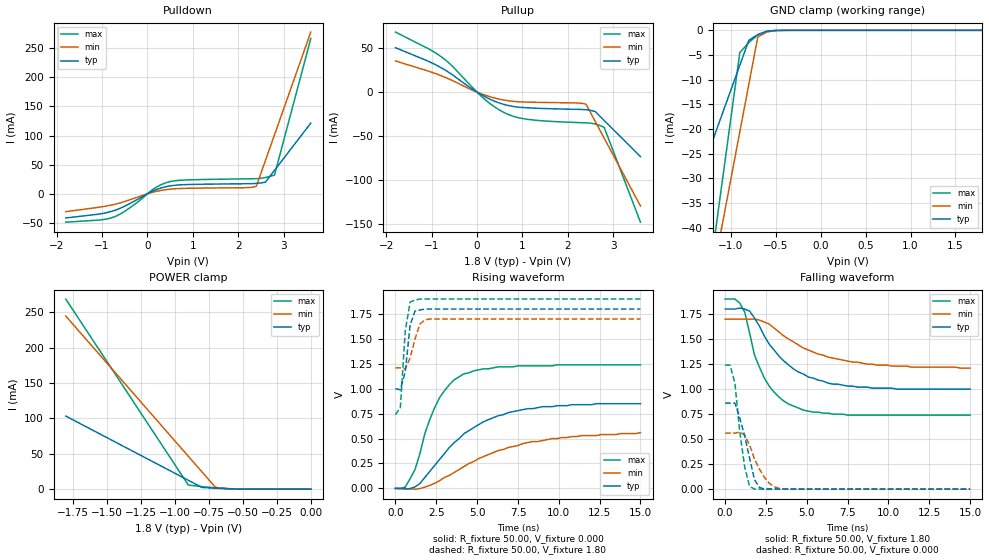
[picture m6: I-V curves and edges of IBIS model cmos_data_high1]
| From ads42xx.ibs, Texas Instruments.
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|   Model cmos_data_high1
[Model]   cmos_data_high1
Model_type   3-state
Polarity   Non-Inverting
Vmeas = 1.0000V
Enable   Active-High
C_comp   5.00pF   2.00pF   8.00pF
[Temperature Range]   25.00   0.12k   -40.00
[Voltage Range]   1.80V   1.70V   1.90V
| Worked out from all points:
|   slope of the pulldown table from 0 to 0.27 V, typ, clamps not added: 29.2 ohm
|   slope of the pullup table from 0 to 0.27 V, typ, clamps not added: 35.5 ohm
|   GND clamp passes 1 mA (typ) near -0.71 V on its own axis
|   POWER clamp passes 1 mA (typ) near -0.67 V on its own axis
|   rising waveform, R_fixture 50.00, V_fixture 0.000: 20-80 % time 3.45ns typ, 4.74ns min, 1.75ns max; typ from 0 V to 0.85 V
|   rising waveform, R_fixture 50.00, V_fixture 1.80: 20-80 % time 317ps typ, 509ps min, 328ps max; typ from 1 V to 1.8 V
|   falling waveform, R_fixture 50.00, V_fixture 1.80: 20-80 % time 2.59ns typ, 3.6ns min, 1.64ns max; typ from 1.8 V to 1 V
|   falling waveform, R_fixture 50.00, V_fixture 0.000: 20-80 % time 755ps typ, 964ps min, 534ps max; typ from 0.86 V to 0 V
[Pulldown]
| voltage   I(typ)   I(min)   I(max)
-1.8V     -41.57mA   -30.74mA   -48.79mA
-1V       -34mA      -22.32mA   -44.53mA
-700mV    -27.96mA   -17.7mA    -38.73mA
-400mV    -17.21mA   -10.58mA   -24.77mA
200mV     7.39mA     4.22mA     11.56mA
500mV     13.57mA    7.94mA     20.94mA
900mV     15.87mA    9.45mA     23.85mA
2.2V      17.23mA    10.57mA    25.67mA
2.4V      17.81mA    12.94mA    25.96mA
2.6V      19.98mA    57.06mA    27.9mA
2.8V      40.26mA    101.2mA    32.1mA
3.6V      121.4mA    277.7mA    266.5mA
[Pullup]
| voltage   I(typ)   I(min)   I(max)
-1.8V     50.62mA    35.54mA    68.37mA
-800mV    28.07mA    18.87mA    40.65mA
-600mV    21.79mA    14.59mA    32.3mA
100mV     -3.08mA    -2mA       -4.97mA
400mV     -10.55mA   -6.83mA    -17.27mA
600mV     -14.02mA   -9.04mA    -23.26mA
800mV     -16.26mA   -10.45mA   -27.47mA
1.1V      -17.71mA   -11.24mA   -30.76mA
2.4V      -19.9mA    -13.64mA   -34.86mA
2.6V      -21.9mA    -32.94mA   -36.12mA
2.8V      -32.16mA   -52.24mA   -39.99mA
3.6V      -73.2mA    -129.4mA   -147.8mA
[GND_clamp]
| voltage   I(typ)   I(min)   I(max)
-1.8V     -52.44mA   -107mA     -124.6mA
-1.6V     -42.36mA   -87.76mA   -97.9mA
-1.5V     -37.32mA   -78.16mA   -84.56mA
-1.2V     -22.2mA    -49.36mA   -44.54mA
-1.1V     -17.16mA   -39.76mA   -31.2mA
-1V       -12.12mA   -30.16mA   -17.86mA
-900mV    -7.08mA    -20.56mA   -4.52mA
-800mV    -2.04mA    -10.96mA   -2.47mA
-700mV    -860uA     -1.36mA    -940uA
-600mV    -210uA     -340uA     -160uA
-400mV    -1.56uA    -9.52uA    -280nA
1.8V      21.86pA    20.03nA    16.21pA
[POWER_clamp]
| voltage   I(typ)   I(min)   I(max)
-1.8V     103.3mA    244.7mA    268.7mA
-900mV    12.58mA    46.54mA    5.82mA
-800mV    2.5mA      24.52mA    3.54mA
-700mV    1.23mA     2.5mA      1.83mA
-500mV    85.21uA    200uA      92.55uA
0V        21.86pA    600pA      19.03pA
[Ramp]
| variable   typ   min   max
dV/dt_r   0.51/3.46n   0.33/4.59n   0.74/1.80n
dV/dt_f   0.48/2.61n   0.29/3.51n   0.70/1.72n
R_load = 50.00
[Rising Waveform]
R_fixture = 50.00
V_fixture = 0.000
V_fixture_min = 0.000
V_fixture_max = 0.000
| time   V(typ)   V(min)   V(max)
0s        -3.27uV    3.72uV     -30.78uV
600ps     -6.61mV    -330uV     13.44mV
1.2ns     15.29mV    -7.79mV    190mV
1.8ns     110mV      12.78mV    550mV
2.7ns     290mV      76.68mV    910mV
3.6ns     460mV      160mV      1.09V
4.2ns     550mV      220mV      1.15V
6.3ns     730mV      380mV      1.22V
8.1ns     800mV      460mV      1.23V
15ns      850mV      560mV      1.24V
[Rising Waveform]
R_fixture = 50.00
V_fixture = 1.80
V_fixture_min = 1.70
V_fixture_max = 1.90
| time   V(typ)   V(min)   V(max)
0s        1V         1.21V      740mV
300ps     990mV      1.21V      810mV
600ps     1.17V      1.2V       1.58V
900ps     1.64V      1.31V      1.87V
1.2ns     1.78V      1.5V       1.89V
1.5ns     1.79V      1.65V      1.9V
1.8ns     1.8V       1.69V      1.9V
2.1ns     1.8V       1.7V       1.9V
15ns      1.8V       1.7V       1.9V
[Falling Waveform]
R_fixture = 50.00
V_fixture = 1.80
V_fixture_min = 1.70
V_fixture_max = 1.90
| time   V(typ)   V(min)   V(max)
0s        1.8V       1.7V       1.9V
900ps     1.81V      1.7V       1.86V
1.2ns     1.8V       1.7V       1.77V
1.5ns     1.78V      1.7V       1.56V
1.8ns     1.71V      1.7V       1.34V
2.4ns     1.53V      1.67V      1.11V
3.9ns     1.24V      1.5V       850mV
5.1ns     1.12V      1.39V      780mV
7.5ns     1.03V      1.28V      740mV
15ns      1V         1.21V      740mV
[Falling Waveform]
R_fixture = 50.00
V_fixture = 0.000
V_fixture_min = 0.000
V_fixture_max = 0.000
| time   V(typ)   V(min)   V(max)
0s        860mV      560mV      1.24V
300ps     860mV      560mV      1.24V
600ps     860mV      560mV      1.06V
900ps     710mV      570mV      570mV
1.2ns     530mV      540mV      220mV
1.5ns     310mV      440mV      27.04mV
1.8ns     93.87mV    300mV      990uV
2.7ns     310uV      59.84mV    320uV
3.3ns     830uV      8.23mV     160uV
15ns      730nV      7.16uV     23.9nV
